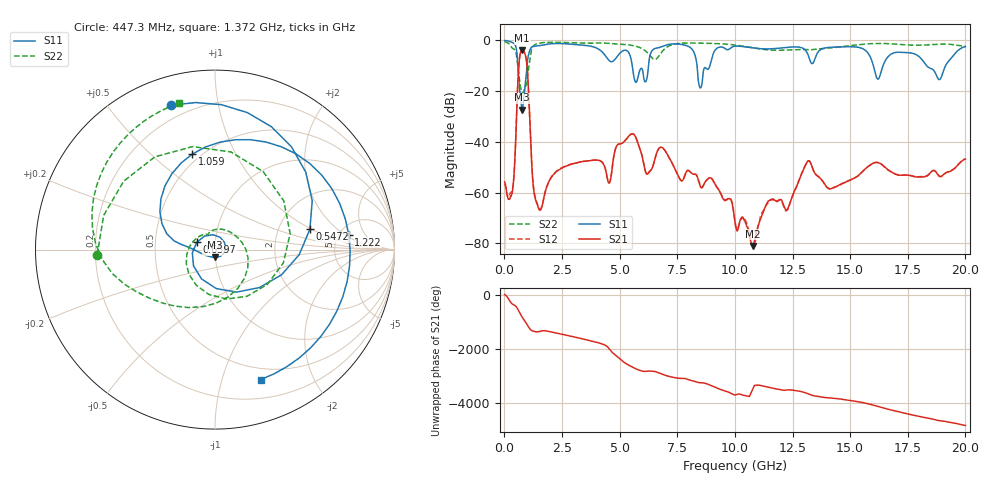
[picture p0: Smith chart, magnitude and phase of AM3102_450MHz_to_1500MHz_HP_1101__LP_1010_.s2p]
!Agilent Technologies,E8364B,MY43040894,A.07.50.67
!Agilent E8364B: A.07.50.67
!Date: Thursday, January 11, 2018 06:39:53
!Correction: S11(Full 2 Port(1,2))
!S21(Full 2 Port(1,2))
!S12(Full 2 Port(1,2))
!S22(Full 2 Port(1,2))
!S2P File: Measurements: S11, S21, S12, S22:
# Hz S  dB  R 50
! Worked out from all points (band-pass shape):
!   1601 points, 10 MHz to 20 GHz, reference 50 ohm
!   highest |S21| = -3.96 dB at 772.1 MHz (marker M1); lowest = -81.0 dB at 10.77 GHz (marker M2)
!   |S21| within 3 dB of the highest: 657.9 MHz to 938.6 MHz (280.7 MHz wide, 35.2 % of centre)
!   lowest |S11| = -27.3 dB at 772.1 MHz (marker M3), VSWR 1.09, Z = 49.7 - j4.27 ohm
!   |S11| at or under -10 dB: 5.548 GHz to 6.25 GHz (702.2 MHz wide, 11.9 % of centre); 8.358 GHz to 8.915 GHz (557.3 MHz wide, 6.45 % of centre); 18.32 GHz to 19.14 GHz (822 MHz wide, 4.39 % of centre)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
!   |S22| runs from -20.8 to -0.5 dB; largest |S21 - S12| = 0.00065
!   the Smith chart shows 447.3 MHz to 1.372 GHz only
!   S11 on the Smith chart (normalised r, x): 447.3 MHz: 0.13, +0.73; 547.2 MHz: 3.01, +0.97; 659.7 MHz: 0.81, +0.07; 1.059 GHz: 0.45, +0.69; 1.222 GHz: 6.08, +2.33; 1.372 GHz: 0.38, -1.34
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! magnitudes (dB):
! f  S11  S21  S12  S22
! 10 MHz  -0.1  -55.7  -56.5  -0.5
! 272.4 MHz  -0.6  -61.3  -59.9  -2.3
! 447.3 MHz  -1.5  -48.6  -48.4  -3.6
! 547.2 MHz  -5.3  -24.6  -24.6  -7.4
! 659.7 MHz  -19.2  -6.8  -6.8  -16.0
! 772.1 MHz  -27.3  -4.0  -4.0  -20.6
! 1.059 GHz  -5.2  -22.0  -22.0  -10.5
! 1.222 GHz  -2.5  -54.0  -53.9  -2.7
! 1.372 GHz  -2.3  -63.3  -62.9  -1.5
! 3.346 GHz  -1.9  -47.8  -47.8  -1.1
! 4.545 GHz  -8.0  -56.2  -56.1  -1.2
! 5.707 GHz  -16.6  -38.4  -38.4  -2.4
! 6.194 GHz  -14.5  -52.8  -52.8  -4.8
! 6.682 GHz  -2.9  -42.9  -42.9  -6.5
! 8.081 GHz  -3.0  -52.0  -52.0  -1.1
! 8.493 GHz  -18.7  -57.4  -57.3  -1.1
! 10.01 GHz  -2.3  -71.7  -71.3  -1.9
! 10.77 GHz  -3.0  -81.0  -80.7  -2.9
! 13.34 GHz  -9.2  -49.6  -49.6  -3.7
! 16.68 GHz  -6.2  -51.2  -51.3  -1.3
! 18.88 GHz  -15.5  -53.6  -53.5  -1.5
! 20 GHz  -2.5  -46.8  -46.7  -2.4
